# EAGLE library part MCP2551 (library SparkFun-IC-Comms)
MCP2551 High Speed CAN Transceiver High speed CAN transceiver Datasheet SparkFun Products CAN-BUS Shield (DEV-13262) SparkFun OBD-II UART (WIG-09555)
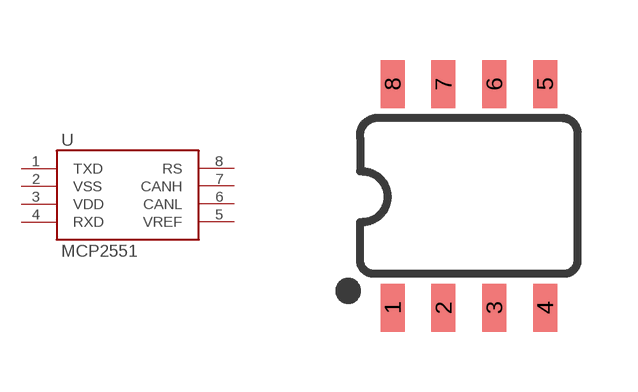
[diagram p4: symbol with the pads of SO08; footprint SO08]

Designator prefix U

## MCP2551 (PROD_ID: IC-09907; VALUE: MCP2551)  [SO08]
1  TXD
2  VSS
3  VDD
4  RXD
5  VREF
6  CANL
7  CANH
8  RS

## Footprint SO08 (pad centres in mm)
SOIC -8 Specifications: Pin count: 8 Width: 0.15" Example device(s): MCP2551
smd 0.6 x 1.2: 1 -1.905,-2.8; 2 -0.635,-2.8; 3 0.635,-2.8; 4 1.905,-2.8; 5 1.905,2.8; 6 0.635,2.8; 7 -0.635,2.8; 8 -1.905,2.8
